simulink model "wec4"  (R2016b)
settings: Solver=ode4  StartTime=0  StopTime=1000  FixedStep=0.005  MaxStep=0.005  RelTol=1e-3  EnableMultiTasking=on
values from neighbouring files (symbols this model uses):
  arAdaptiveLawData = 1/2*zModelSimple.zModelPto.arFreq.*     zModelSimple.zModelPto.arMagnitude./     cos(zModelSimple.zModelPto.arPhase*pi/180+pi/2)    [IMPACT_Control.m]
  arAdaptiveLawDataX = 1/2*zModelSimpleX.zModelPto.arFreq.*         zModelSimpleX.zModelPto.arMagnitude./         cos(zModelSimpleX.zModelPto.arPhase*pi/180+pi/2)    [IMPACT_Control.m]
  arControllerRampGain = [0,0,1,1]    [IMPACT_Control.m]
  arControllerRampTime = [0 rStartRampTime rStartRampTime+rRampTimeLength 8000]    [IMPACT_Control.m]
  arEkfInitialisation = zeros(1,11)    [IMPACT_Control.m]
  arEkfInitialisationX = zeros(1,11)    [IMPACT_Control.m]
  arFrequency = zModelSimple.zModelPto.arFreq    [IMPACT_Control.m]
  arFrequencyRange = zModelSimple.zModelPto.arFreq    [IMPACT_Control.m]
  arFrequencyX = zModelSimpleX.zModelPto.arFreq    [IMPACT_Control.m]
  arImpedance = 1./zModelSimple.zModelPto.arMagnitude./zModelSimple.zModelPto.arFreq    [IMPACT_Control.m]
  arImpedanceX = 1./zModelSimpleX.zModelPto.arMagnitude./zModelSimpleX.zModelPto.arFreq    [IMPACT_Control.m]
  CentralPTOPreload = -1.6113e+07    (= -16113000)    [wecSimInputFile.m]
  F1 = [4.243 2.375 -12.243]    [wecSimInputFile.m]
  F2 = [4.243 -2.375 -12.243]    [wecSimInputFile.m]
  F3 = [-4.243 -2.375 -12.243]    [wecSimInputFile.m]
  F4 = [-4.243 2.375 -12.243]    [wecSimInputFile.m]
  FC = [0 0 -14]    [wecSimInputFile.m]
  iAdaptiveDamping = 0    [wec4IMPACT_Project.m]    (also in IMPACT_Control.m = handles.iAdaptiveDamping; wec1_IMPACT_Project.m; wec2_IMPACT_Project.m; wec3_IMPACT_Project.m)
  iControlType = 2    [wec4IMPACT_Project.m]    (also in IMPACT_Control.m = handles.iControlType; wec1_IMPACT_Project.m = 1; wec2_IMPACT_Project.m = 1; wec3_IMPACT_Project.m = 1)
  iPtoPositionConstraint = 1    [wec4IMPACT_Project.m]    (also in IMPACT_Control.m = handles.iPtoPositionConstraint; wec1_IMPACT_Project.m = 0; wec2_IMPACT_Project.m; wec3_IMPACT_Project.m)
  iSensorNoise = 0    [IMPACT_Control.m]
  m = m+1    (= 2)    [checkParamFile.m]
  PTOrotation = atan((T1(2)-F1(2))/(T1(1)-F1(1)))    [wecSimInputFile.m]
  rCogFloater = -8    [wec4_IMPACT_Model.m]    (also in paramInitial.m = get( handles.edit_rCogFloater, 'String' ); wec1_IMPACT_Model.m = -18; wec2_IMPACT_Model.m = -8.5; wec3_IMPACT_Model.m = -0.7)
  rCogSpar = -36.6    [wec4_IMPACT_Model.m]    (also in paramInitial.m = get( handles.edit_rCogSpar, 'String' ); wec3_IMPACT_Model.m = -21.3; wec3_IMPACT_Model2.m = -21.3)
  rDisplacementLimit = 10.000000    (= 10)    [wec4IMPACT_Project.m]    (also in IMPACT_Control.m = getValue(handles.edit_displacementLimit); wec1_IMPACT_Project.m; wec2_IMPACT_Project.m; wec3_IMPACT_Project.m = 3)
  rDisplacementLimitX = 10.000000    (= 10)    [wec4IMPACT_Project.m]    (also in IMPACT_Control.m = getValue(handles.edit_displacementLimitX); wec1_IMPACT_Project.m = 0; wec2_IMPACT_Project.m; wec3_IMPACT_Project.m = 0)
  rGainForAntiWIndUp = tfControllerDiscrete.rGain    [IMPACT_Control.m]
  rGainForAntiWIndUpX = tfControllerXDiscrete.rGain    [IMPACT_Control.m]
  rMaxForcePto = 300000000.000000    (= 300000000)    [wec4IMPACT_Project.m]    (also in IMPACT_Control.m = getValue(handles.edit_maxForcePto); wec1_IMPACT_Project.m = 1e+15; wec2_IMPACT_Project.m = 1e+15; wec3_IMPACT_Project.m = 1000000000)
  rMinForcePto = -300000000.000000    (= -300000000)    [wec4IMPACT_Project.m]    (also in IMPACT_Control.m = getValue(handles.edit_minForcePto); wec1_IMPACT_Project.m = -1e+15; wec2_IMPACT_Project.m = -1e+15; wec3_IMPACT_Project.m = -1000000000)
  rMooringX = 20000    [wec4_IMPACT_Model.m]    (also in paramInitial.m = get( handles.edit_rMooringX, 'String' ); wec3_IMPACT_Model.m = 10000; wec3_IMPACT_Model2.m = 10000)
  rMooringZ = 10000    [wec4_IMPACT_Model.m]    (also in paramInitial.m = get( handles.edit_rMooringZ, 'String' ); wec3_IMPACT_Model.m = 0; wec3_IMPACT_Model2.m = 0)
  rOutputSampleTime = 0.010000    (= 0.01)    [wec4IMPACT_Project.m]    (also in IMPACT_Control.m = getValue(handles.edit_outputSampleTime); wec1_IMPACT_Project.m; wec2_IMPACT_Project.m; wec3_IMPACT_Project.m)
  rPassiveDampingGain = -604830.000000    (= -604830)    [wec4IMPACT_Project.m]    (also in IMPACT_Control.m = getValue(handles.edit_gainPLD); wec1_IMPACT_Project.m = -214018.1537; wec2_IMPACT_Project.m = -1948070; wec3_IMPACT_Project.m = -519390)
  rPassiveDampingGainX = -278660.000000    (= -278660)    [wec4IMPACT_Project.m]    (also in IMPACT_Control.m = getValue(handles.edit_gainPLDX); wec1_IMPACT_Project.m = 0; wec2_IMPACT_Project.m = 0; wec3_IMPACT_Project.m = 0)
  rTetherPretension = 1.6113e+07    (= 16113000)    [wec4_IMPACT_Model.m]    (also in paramInitial.m = get( handles.edit_rTetherPretension, 'String' ); wec3_IMPACT_Model.m = 0; wec3_IMPACT_Model2.m = 0)
  rTetherSpring = 500000    [wec4_IMPACT_Model.m]    (also in paramInitial.m = get( handles.edit_rTetherSpring, 'String' ); wec3_IMPACT_Model.m = 0; wec3_IMPACT_Model2.m = 0)
  rUpperFrequencyLimit = EKFFloater.upperFreq    [IMPACT_Control.m]
  rXf = 4.243    [wec4AdditionalParams.m]
  rXs = 16.075    [wec4AdditionalParams.m]
  rYf = 2.375    [wec4AdditionalParams.m]
  rYs = 16.075    [wec4AdditionalParams.m]
  rZf = 4.243    [wec4AdditionalParams.m]
  rZs = 2.4350    (= 2.435)    [wec4AdditionalParams.m]
  rZTetherF = 6    [wec4AdditionalParams.m]
  rZTetherS = 2.4350    (= 2.435)    [wec4AdditionalParams.m]
  s = tf('s')    [wec4_IMPACT_Model.m]    (also in IMPACT_Control.m; wec1_IMPACT_Model.m; wec2_IMPACT_Model.m; wec3_IMPACT_Model.m)
  SidePTO1Preload = PreloadPTOCorner    (= 0)    [wecSimInputFile.m]
  SidePTO2Preload = PreloadPTOCorner    (= 0)    [wecSimInputFile.m]
  SidePTO3Preload = PreloadPTOCorner    (= 0)    [wecSimInputFile.m]
  SidePTO4Preload = PreloadPTOCorner    (= 0)    [wecSimInputFile.m]
  simu = simulationClass()    [wecSimInputFile.m]
  T1 = [16.075 16.075 -34.165]    [wecSimInputFile.m]
  T2 = [16.075 -16.075 -34.165]    [wecSimInputFile.m]
  T3 = [-16.075 -16.075 -34.165]    [wecSimInputFile.m]
  T4 = [-16.075 16.075 -34.165]    [wecSimInputFile.m]
  TC = [0 0 -34.165]    [wecSimInputFile.m]
  waves = waveClass('irregular')    [wecSimInputFile.m]
  Z = magPhaseToComplex(zModelTf)    [IMPACT_Control.m]
undefined symbols (not defined in the file or in its folder): arControllerDiscreteDen, arControllerDiscreteNum, arControllerDiscreteXDen, arControllerDiscreteXNum, arExcForceFloaterDen, arExcForceFloaterNum, arExcForceFloaterXDen, arExcForceFloaterXNum, arExcForceSparDen, arExcForceSparNum, arExcForceSparXDen, arExcForceSparXNum, arFexcFloaterDen, arFexcFloaterNum, arFexcFloaterXDen, arFexcFloaterXNum, arFexcSparDen, arFexcSparNum, arFexcSparXDen, arFexcSparXNum, Body, body, constraint, CTTime, deg, Elements, geometry, IRKB, kg, lenJ, mooring, N, pto, rAccelerationGainFloater, rAccelerationGainFloaterX, rAccelerationGainSpar, rAccelerationGainSparX, rad, rBuoyancyGainFloater, rBuoyancyGainFloaterX, rBuoyancyGainSpar, rBuoyancyGainSparX, rDampingGainFloater, rDampingGainFloaterX, rDampingGainSpar, rDampingGainSparX, Rigid, rMaxFocePto, wec4_float, wec4_reactor, WECSim_Lib, X, Y
libraries: nesl_utility x380, sm_lib x170, vrlib x91, simulink x12, WECSim_Lib x4
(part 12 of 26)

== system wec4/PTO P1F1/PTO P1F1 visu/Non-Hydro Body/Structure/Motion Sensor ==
  note: Measures the position, velocity, and acceleration of the follower (F) frame relative to the base (B) frame. Ouputs a bus of 3 signals, each signal is a vector length 6.
  Angle : MATLAB Function  TreatAsAtomicUnit=on
  Bus Creator : BusCreator  Inputs=3
  Mux : Mux
  Mux1 : Mux  Inputs=6
  Mux2 : Mux  Inputs=6
  PS-Simulink Converter{,1..15} (16 alike) : nesl_utility/PS-Simulink Converter  PhysicalDomain=network_engine_domain  SubClassName=ps_output  LeftPortType=input  RightPortType=output  PseudoPeriodic=off  Frequencies=[]  Unit=1  AffineConversion=off
  Transform Sensor : sm_lib/Frames and Transforms/Transform Sensor  MeasurementFrame=World  SenseAngle=off  SenseAxis=off  SenseAngle1=off  SenseAngle2=off  SenseAngle3=off  SenseQ=on  SenseR=off  SenseOmegaX=on  SenseOmegaY=on  SenseOmegaZ=on  SenseOmega1=off  SenseOmega2=off  SenseOmega3=off  SenseQDot=off  SenseRDot=off  SenseAlphaX=on  SenseAlphaY=on  SenseAlphaZ=on  SenseAlpha1=off  SenseAlpha2=off  SenseAlpha3=off  SenseQDDot=off  SenseRDDot=off  SenseX=on  SenseY=on  SenseZ=on  SenseRad=off  SenseAzim=off  SenseDist=off  SenseInc=off  SenseXDot=on  SenseYDot=on  SenseZDot=on  SenseRadDot=off  SenseAzimDot=off  SenseDistDot=off  SenseIncDot=off  SenseXDDot=on  SenseYDDot=on  SenseZDDot=on  SenseRadDDot=off  SenseAzimDDot=off  SenseDistDDot=off  SenseIncDDot=off
  F : PMIOPort  Port=1  Side=Right
  B : PMIOPort  Port=2  Side=Left
  Response : Outport
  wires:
  PS-Simulink Converter/1 -> Angle/1(Q)
  PS-Simulink Converter4/1 -> Mux2/4  "alphax"
  PS-Simulink Converter10/1 -> Mux1/1  "vx"
  PS-Simulink Converter12/1 -> Mux1/3  "vz"
  PS-Simulink Converter13/1 -> Mux2/1  "ax"
  PS-Simulink Converter14/1 -> Mux2/2  "ay"
  Mux/1 -> Bus Creator/1  "disp"
  Mux1/1 -> Bus Creator/2  "vel"
  Mux2/1 -> Bus Creator/3  "acc"
  Angle/1(E) -> Mux/4
  PS-Simulink Converter7/1 -> Mux/1  "x"
  PS-Simulink Converter8/1 -> Mux/2  "y"
  PS-Simulink Converter9/1 -> Mux/3  "z"
  PS-Simulink Converter5/1 -> Mux2/5  "alphay"
  PS-Simulink Converter6/1 -> Mux2/6  "alphaz"
  PS-Simulink Converter1/1 -> Mux1/4  "omegax"
  PS-Simulink Converter2/1 -> Mux1/5  "omegay"
  PS-Simulink Converter11/1 -> Mux1/2  "vy"
  PS-Simulink Converter3/1 -> Mux1/6  "omegaz"
  PS-Simulink Converter15/1 -> Mux2/3  "az"
  Bus Creator/1 -> Response/1
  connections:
  Transform Sensor/RConn1 -- F/RConn1
  B/RConn1 -- Transform Sensor/LConn1
  Transform Sensor/RConn2 -- PS-Simulink Converter/LConn1
  PS-Simulink Converter15/LConn1 -- Transform Sensor/RConn17
  PS-Simulink Converter14/LConn1 -- Transform Sensor/RConn16
  PS-Simulink Converter13/LConn1 -- Transform Sensor/RConn15
  PS-Simulink Converter12/LConn1 -- Transform Sensor/RConn14
  PS-Simulink Converter11/LConn1 -- Transform Sensor/RConn13
  PS-Simulink Converter10/LConn1 -- Transform Sensor/RConn12
  PS-Simulink Converter9/LConn1 -- Transform Sensor/RConn11
  PS-Simulink Converter8/LConn1 -- Transform Sensor/RConn10
  PS-Simulink Converter7/LConn1 -- Transform Sensor/RConn9
  PS-Simulink Converter4/LConn1 -- Transform Sensor/RConn6
  PS-Simulink Converter5/LConn1 -- Transform Sensor/RConn7
  PS-Simulink Converter6/LConn1 -- Transform Sensor/RConn8
  PS-Simulink Converter1/LConn1 -- Transform Sensor/RConn3
  PS-Simulink Converter2/LConn1 -- Transform Sensor/RConn4
  PS-Simulink Converter3/LConn1 -- Transform Sensor/RConn5

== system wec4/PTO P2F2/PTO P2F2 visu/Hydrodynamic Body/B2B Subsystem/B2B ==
  CrossCoupling : Subsystem
  vel : Outport
  acc : Outport  Port=2
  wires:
  CrossCoupling/2(acc) -> acc/1
  CrossCoupling/1(vel) -> vel/1

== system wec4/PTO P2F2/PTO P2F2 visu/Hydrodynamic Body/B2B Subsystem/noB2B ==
  vel_in : Inport
  acc_in : Inport  Port=2
  vel : Outport
  acc : Outport  Port=2
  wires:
  acc_in/1 -> acc/1
  vel_in/1 -> vel/1  "x"

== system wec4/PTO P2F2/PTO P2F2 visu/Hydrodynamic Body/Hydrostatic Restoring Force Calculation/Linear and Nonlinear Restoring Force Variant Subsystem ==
  note: 1) Add Subsystem or Model blocks as valid variant choices. 2) You cannot connect blocks at this level. At simulation, connectivity is automatically determined, based on the active variant and port name matching.
  In1 : Inport
  In2 : Inport  Port=2
  "Linear Hydrostatic Restoring Force " : Subsystem  VariantControl=sv_linearHydro
  Nonlinear Hydrostatic Restoring Force : Subsystem  VariantControl=sv_nonlinearHydro
  Out1 : Outport

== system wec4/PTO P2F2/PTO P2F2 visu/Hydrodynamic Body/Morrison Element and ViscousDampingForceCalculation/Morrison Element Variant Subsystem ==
  note: 1) Add Subsystem or Model blocks as valid variant choices. 2) You cannot connect blocks at this level. At simulation, connectivity is automatically determined, based on the active variant and port name matching.
  displacement : Inport
  velocity : Inport  Port=2
  acceleration : Inport  Port=3
  time : Inport  Port=4
  Morrison Element Off : Subsystem  VariantControl=sv_MEOff
  Morrison Element On : Subsystem  Variant=on  VariantControl=sv_MEOn
  morison_force : Outport

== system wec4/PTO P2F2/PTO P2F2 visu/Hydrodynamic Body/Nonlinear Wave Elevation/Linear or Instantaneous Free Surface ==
  note: 1) Add Subsystem or Model blocks as valid variant choices. 2) You cannot connect blocks at this level. At simulation, connectivity is automatically determined, based on the active variant and port name matching.
  In1 : Inport
  In2 : Inport  Port=2
  "Instantaneous Water Free Surface  " : Subsystem  VariantControl=sv_instFS
  "Mean Water Free Surface " : Subsystem  VariantControl=sv_meanFS
  Out1 : Outport

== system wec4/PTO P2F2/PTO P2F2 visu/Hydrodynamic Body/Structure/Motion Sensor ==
  note: Measures the position, velocity, and acceleration of the follower (F) frame relative to the base (B) frame. Ouputs a bus of 3 signals, each signal is a vector length 6.
  Angle : MATLAB Function  TreatAsAtomicUnit=on
  Bus Creator : BusCreator  Inputs=3
  Mux : Mux
  Mux1 : Mux  Inputs=6
  Mux2 : Mux  Inputs=6
  PS-Simulink Converter{,1..15} (16 alike) : nesl_utility/PS-Simulink Converter  PhysicalDomain=network_engine_domain  SubClassName=ps_output  LeftPortType=input  RightPortType=output  PseudoPeriodic=off  Frequencies=[]  Unit=1  AffineConversion=off
  Transform Sensor : sm_lib/Frames and Transforms/Transform Sensor  MeasurementFrame=World  SenseAngle=off  SenseAxis=off  SenseAngle1=off  SenseAngle2=off  SenseAngle3=off  SenseQ=on  SenseR=off  SenseOmegaX=on  SenseOmegaY=on  SenseOmegaZ=on  SenseOmega1=off  SenseOmega2=off  SenseOmega3=off  SenseQDot=off  SenseRDot=off  SenseAlphaX=on  SenseAlphaY=on  SenseAlphaZ=on  SenseAlpha1=off  SenseAlpha2=off  SenseAlpha3=off  SenseQDDot=off  SenseRDDot=off  SenseX=on  SenseY=on  SenseZ=on  SenseRad=off  SenseAzim=off  SenseDist=off  SenseInc=off  SenseXDot=on  SenseYDot=on  SenseZDot=on  SenseRadDot=off  SenseAzimDot=off  SenseDistDot=off  SenseIncDot=off  SenseXDDot=on  SenseYDDot=on  SenseZDDot=on  SenseRadDDot=off  SenseAzimDDot=off  SenseDistDDot=off  SenseIncDDot=off
  F : PMIOPort  Port=1  Side=Right
  B : PMIOPort  Port=2  Side=Left
  Response : Outport
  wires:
  PS-Simulink Converter/1 -> Angle/1(Q)
  PS-Simulink Converter4/1 -> Mux2/4  "alphax"
  PS-Simulink Converter10/1 -> Mux1/1  "vx"
  PS-Simulink Converter12/1 -> Mux1/3  "vz"
  PS-Simulink Converter13/1 -> Mux2/1  "ax"
  PS-Simulink Converter14/1 -> Mux2/2  "ay"
  Mux/1 -> Bus Creator/1  "disp"
  Mux1/1 -> Bus Creator/2  "vel"
  Mux2/1 -> Bus Creator/3  "acc"
  Angle/1(E) -> Mux/4
  PS-Simulink Converter7/1 -> Mux/1  "x"
  PS-Simulink Converter8/1 -> Mux/2  "y"
  PS-Simulink Converter9/1 -> Mux/3  "z"
  PS-Simulink Converter5/1 -> Mux2/5  "alphay"
  PS-Simulink Converter6/1 -> Mux2/6  "alphaz"
  PS-Simulink Converter1/1 -> Mux1/4  "omegax"
  PS-Simulink Converter2/1 -> Mux1/5  "omegay"
  PS-Simulink Converter11/1 -> Mux1/2  "vy"
  PS-Simulink Converter3/1 -> Mux1/6  "omegaz"
  PS-Simulink Converter15/1 -> Mux2/3  "az"
  Bus Creator/1 -> Response/1
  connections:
  Transform Sensor/RConn1 -- F/RConn1
  B/RConn1 -- Transform Sensor/LConn1
  Transform Sensor/RConn2 -- PS-Simulink Converter/LConn1
  PS-Simulink Converter15/LConn1 -- Transform Sensor/RConn17
  PS-Simulink Converter14/LConn1 -- Transform Sensor/RConn16
  PS-Simulink Converter13/LConn1 -- Transform Sensor/RConn15
  PS-Simulink Converter12/LConn1 -- Transform Sensor/RConn14
  PS-Simulink Converter11/LConn1 -- Transform Sensor/RConn13
  PS-Simulink Converter10/LConn1 -- Transform Sensor/RConn12
  PS-Simulink Converter9/LConn1 -- Transform Sensor/RConn11
  PS-Simulink Converter8/LConn1 -- Transform Sensor/RConn10
  PS-Simulink Converter7/LConn1 -- Transform Sensor/RConn9
  PS-Simulink Converter4/LConn1 -- Transform Sensor/RConn6
  PS-Simulink Converter5/LConn1 -- Transform Sensor/RConn7
  PS-Simulink Converter6/LConn1 -- Transform Sensor/RConn8
  PS-Simulink Converter1/LConn1 -- Transform Sensor/RConn3
  PS-Simulink Converter2/LConn1 -- Transform Sensor/RConn4
  PS-Simulink Converter3/LConn1 -- Transform Sensor/RConn5

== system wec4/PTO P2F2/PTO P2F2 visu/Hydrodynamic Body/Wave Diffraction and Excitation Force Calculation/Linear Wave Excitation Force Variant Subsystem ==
  note: 1) Add Subsystem or Model blocks as valid variant choices. 2) You cannot connect blocks at this level. At simulation, connectivity is automatically determined, based on the active variant and port name matching.
  In1 : Inport
  Irregular Wave Excitation Force : Subsystem  VariantControl=sv_irregularWaves
  No Wave Excitation Force : Subsystem  VariantControl=sv_noWave
  Regular Wave Excitation Force : Subsystem  VariantControl=sv_regularWaves
  User Defined Wave Excitation Force : Subsystem  VariantControl=sv_udfWaves
  Out1 : Outport

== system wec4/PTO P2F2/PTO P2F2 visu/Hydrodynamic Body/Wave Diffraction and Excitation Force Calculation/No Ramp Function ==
  Action Port : ActionPort
  Constant : Constant
  R : Outport  InitialOutput=1
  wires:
  Constant/1 -> R/1

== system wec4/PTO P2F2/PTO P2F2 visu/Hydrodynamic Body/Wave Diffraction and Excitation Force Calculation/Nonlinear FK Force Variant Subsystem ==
  note: 1) Add Subsystem or Model blocks as valid variant choices. 2) You cannot connect blocks at this level. At simulation, connectivity is automatically determined, based on the active variant and port name matching.
  In1 : Inport
  In2 : Inport  Port=2
  In3 : Inport  Port=3
  No Nonlinear FroudeKrylov Force : Subsystem  VariantControl=sv_linearHydro
  With Nonlinear FroudeKrylov Force : Subsystem  TreatAsAtomicUnit=on  SystemSampleTime=simu.dtNL  VariantControl=sv_nonlinearHydro
  Out1 : Outport

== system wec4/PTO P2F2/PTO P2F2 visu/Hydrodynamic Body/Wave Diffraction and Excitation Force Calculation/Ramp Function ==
  Time : Inport
  Action Port : ActionPort
  Add : Sum
  Add1 : Sum
  Constant : Constant  Value=1/2
  Constant1 : Constant
  Constant2 : Constant  Value=3*pi/2
  Constant3 : Constant  Value=pi
  Divide : Product  Inputs=*/
  Product : Product
  Product1 : Product
  Ramp Time : Constant  Value=simu.rampTime
  Sine Wave Function : Sin  TimeSource=Use external signal  SampleTime=0
  R : Outport
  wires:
  Divide/1 -> Product1/2  "frequency"
  Constant3/1 -> Divide/1
  Product1/1 -> Add1/1
  Add1/1 -> Sine Wave Function/1
  Constant2/1 -> Add1/2  "phase"
  Ramp Time/1 -> Divide/2  "t_ramp"
  Time/1 -> Product1/1  "t"
  Product/1 -> R/1
  Constant/1 -> Product/2
  Constant1/1 -> Add/1
  Sine Wave Function/1 -> Add/2
  Add/1 -> Product/1

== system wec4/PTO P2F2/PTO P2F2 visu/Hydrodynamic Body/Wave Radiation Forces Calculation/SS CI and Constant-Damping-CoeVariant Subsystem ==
  note: 1) Add Subsystem or Model blocks as valid variant choices. 2) You cannot connect blocks at this level. At simulation, connectivity is automatically determined, based on the active variant and port name matching.
  In1 : Inport
  In2 : Inport  Port=2
  Constant Coefficients : Subsystem  VariantControl=sv_constantCoeff
  Convolution Integral Calculation : Subsystem  VariantControl=sv_convolution
  "State-Space Calculation " : Subsystem  VariantControl=sv_stateSpace
  Out1 : Outport

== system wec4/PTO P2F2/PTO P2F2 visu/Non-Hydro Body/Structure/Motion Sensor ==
  note: Measures the position, velocity, and acceleration of the follower (F) frame relative to the base (B) frame. Ouputs a bus of 3 signals, each signal is a vector length 6.
  Angle : MATLAB Function  TreatAsAtomicUnit=on
  Bus Creator : BusCreator  Inputs=3
  Mux : Mux
  Mux1 : Mux  Inputs=6
  Mux2 : Mux  Inputs=6
  PS-Simulink Converter{,1..15} (16 alike) : nesl_utility/PS-Simulink Converter  PhysicalDomain=network_engine_domain  SubClassName=ps_output  LeftPortType=input  RightPortType=output  PseudoPeriodic=off  Frequencies=[]  Unit=1  AffineConversion=off
  Transform Sensor : sm_lib/Frames and Transforms/Transform Sensor  MeasurementFrame=World  SenseAngle=off  SenseAxis=off  SenseAngle1=off  SenseAngle2=off  SenseAngle3=off  SenseQ=on  SenseR=off  SenseOmegaX=on  SenseOmegaY=on  SenseOmegaZ=on  SenseOmega1=off  SenseOmega2=off  SenseOmega3=off  SenseQDot=off  SenseRDot=off  SenseAlphaX=on  SenseAlphaY=on  SenseAlphaZ=on  SenseAlpha1=off  SenseAlpha2=off  SenseAlpha3=off  SenseQDDot=off  SenseRDDot=off  SenseX=on  SenseY=on  SenseZ=on  SenseRad=off  SenseAzim=off  SenseDist=off  SenseInc=off  SenseXDot=on  SenseYDot=on  SenseZDot=on  SenseRadDot=off  SenseAzimDot=off  SenseDistDot=off  SenseIncDot=off  SenseXDDot=on  SenseYDDot=on  SenseZDDot=on  SenseRadDDot=off  SenseAzimDDot=off  SenseDistDDot=off  SenseIncDDot=off
  F : PMIOPort  Port=1  Side=Right
  B : PMIOPort  Port=2  Side=Left
  Response : Outport
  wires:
  PS-Simulink Converter/1 -> Angle/1(Q)
  PS-Simulink Converter4/1 -> Mux2/4  "alphax"
  PS-Simulink Converter10/1 -> Mux1/1  "vx"
  PS-Simulink Converter12/1 -> Mux1/3  "vz"
  PS-Simulink Converter13/1 -> Mux2/1  "ax"
  PS-Simulink Converter14/1 -> Mux2/2  "ay"
  Mux/1 -> Bus Creator/1  "disp"
  Mux1/1 -> Bus Creator/2  "vel"
  Mux2/1 -> Bus Creator/3  "acc"
  Angle/1(E) -> Mux/4
  PS-Simulink Converter7/1 -> Mux/1  "x"
  PS-Simulink Converter8/1 -> Mux/2  "y"
  PS-Simulink Converter9/1 -> Mux/3  "z"
  PS-Simulink Converter5/1 -> Mux2/5  "alphay"
  PS-Simulink Converter6/1 -> Mux2/6  "alphaz"
  PS-Simulink Converter1/1 -> Mux1/4  "omegax"
  PS-Simulink Converter2/1 -> Mux1/5  "omegay"
  PS-Simulink Converter11/1 -> Mux1/2  "vy"
  PS-Simulink Converter3/1 -> Mux1/6  "omegaz"
  PS-Simulink Converter15/1 -> Mux2/3  "az"
  Bus Creator/1 -> Response/1
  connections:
  Transform Sensor/RConn1 -- F/RConn1
  B/RConn1 -- Transform Sensor/LConn1
  Transform Sensor/RConn2 -- PS-Simulink Converter/LConn1
  PS-Simulink Converter15/LConn1 -- Transform Sensor/RConn17
  PS-Simulink Converter14/LConn1 -- Transform Sensor/RConn16
  PS-Simulink Converter13/LConn1 -- Transform Sensor/RConn15
  PS-Simulink Converter12/LConn1 -- Transform Sensor/RConn14
  PS-Simulink Converter11/LConn1 -- Transform Sensor/RConn13
  PS-Simulink Converter10/LConn1 -- Transform Sensor/RConn12
  PS-Simulink Converter9/LConn1 -- Transform Sensor/RConn11
  PS-Simulink Converter8/LConn1 -- Transform Sensor/RConn10
  PS-Simulink Converter7/LConn1 -- Transform Sensor/RConn9
  PS-Simulink Converter4/LConn1 -- Transform Sensor/RConn6
  PS-Simulink Converter5/LConn1 -- Transform Sensor/RConn7
  PS-Simulink Converter6/LConn1 -- Transform Sensor/RConn8
  PS-Simulink Converter1/LConn1 -- Transform Sensor/RConn3
  PS-Simulink Converter2/LConn1 -- Transform Sensor/RConn4
  PS-Simulink Converter3/LConn1 -- Transform Sensor/RConn5

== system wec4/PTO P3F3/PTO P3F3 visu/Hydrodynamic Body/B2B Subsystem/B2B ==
  CrossCoupling : Subsystem
  vel : Outport
  acc : Outport  Port=2
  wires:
  CrossCoupling/2(acc) -> acc/1
  CrossCoupling/1(vel) -> vel/1

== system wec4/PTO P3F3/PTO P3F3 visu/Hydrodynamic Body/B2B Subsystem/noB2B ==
  vel_in : Inport
  acc_in : Inport  Port=2
  vel : Outport
  acc : Outport  Port=2
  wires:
  acc_in/1 -> acc/1
  vel_in/1 -> vel/1  "x"

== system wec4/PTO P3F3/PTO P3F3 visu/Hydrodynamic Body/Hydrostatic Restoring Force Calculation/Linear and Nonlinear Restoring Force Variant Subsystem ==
  note: 1) Add Subsystem or Model blocks as valid variant choices. 2) You cannot connect blocks at this level. At simulation, connectivity is automatically determined, based on the active variant and port name matching.
  In1 : Inport
  In2 : Inport  Port=2
  "Linear Hydrostatic Restoring Force " : Subsystem  VariantControl=sv_linearHydro
  Nonlinear Hydrostatic Restoring Force : Subsystem  VariantControl=sv_nonlinearHydro
  Out1 : Outport

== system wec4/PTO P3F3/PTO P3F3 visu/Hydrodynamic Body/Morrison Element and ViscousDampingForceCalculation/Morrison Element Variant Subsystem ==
  note: 1) Add Subsystem or Model blocks as valid variant choices. 2) You cannot connect blocks at this level. At simulation, connectivity is automatically determined, based on the active variant and port name matching.
  displacement : Inport
  velocity : Inport  Port=2
  acceleration : Inport  Port=3
  time : Inport  Port=4
  Morrison Element Off : Subsystem  VariantControl=sv_MEOff
  Morrison Element On : Subsystem  Variant=on  VariantControl=sv_MEOn
  morison_force : Outport

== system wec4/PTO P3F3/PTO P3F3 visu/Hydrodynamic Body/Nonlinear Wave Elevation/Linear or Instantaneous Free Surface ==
  note: 1) Add Subsystem or Model blocks as valid variant choices. 2) You cannot connect blocks at this level. At simulation, connectivity is automatically determined, based on the active variant and port name matching.
  In1 : Inport
  In2 : Inport  Port=2
  "Instantaneous Water Free Surface  " : Subsystem  VariantControl=sv_instFS
  "Mean Water Free Surface " : Subsystem  VariantControl=sv_meanFS
  Out1 : Outport

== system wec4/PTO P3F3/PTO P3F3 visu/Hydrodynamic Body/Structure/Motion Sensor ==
  note: Measures the position, velocity, and acceleration of the follower (F) frame relative to the base (B) frame. Ouputs a bus of 3 signals, each signal is a vector length 6.
  Angle : MATLAB Function  TreatAsAtomicUnit=on
  Bus Creator : BusCreator  Inputs=3
  Mux : Mux
  Mux1 : Mux  Inputs=6
  Mux2 : Mux  Inputs=6
  PS-Simulink Converter{,1..15} (16 alike) : nesl_utility/PS-Simulink Converter  PhysicalDomain=network_engine_domain  SubClassName=ps_output  LeftPortType=input  RightPortType=output  PseudoPeriodic=off  Frequencies=[]  Unit=1  AffineConversion=off
  Transform Sensor : sm_lib/Frames and Transforms/Transform Sensor  MeasurementFrame=World  SenseAngle=off  SenseAxis=off  SenseAngle1=off  SenseAngle2=off  SenseAngle3=off  SenseQ=on  SenseR=off  SenseOmegaX=on  SenseOmegaY=on  SenseOmegaZ=on  SenseOmega1=off  SenseOmega2=off  SenseOmega3=off  SenseQDot=off  SenseRDot=off  SenseAlphaX=on  SenseAlphaY=on  SenseAlphaZ=on  SenseAlpha1=off  SenseAlpha2=off  SenseAlpha3=off  SenseQDDot=off  SenseRDDot=off  SenseX=on  SenseY=on  SenseZ=on  SenseRad=off  SenseAzim=off  SenseDist=off  SenseInc=off  SenseXDot=on  SenseYDot=on  SenseZDot=on  SenseRadDot=off  SenseAzimDot=off  SenseDistDot=off  SenseIncDot=off  SenseXDDot=on  SenseYDDot=on  SenseZDDot=on  SenseRadDDot=off  SenseAzimDDot=off  SenseDistDDot=off  SenseIncDDot=off
  F : PMIOPort  Port=1  Side=Right
  B : PMIOPort  Port=2  Side=Left
  Response : Outport
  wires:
  PS-Simulink Converter/1 -> Angle/1(Q)
  PS-Simulink Converter4/1 -> Mux2/4  "alphax"
  PS-Simulink Converter10/1 -> Mux1/1  "vx"
  PS-Simulink Converter12/1 -> Mux1/3  "vz"
  PS-Simulink Converter13/1 -> Mux2/1  "ax"
  PS-Simulink Converter14/1 -> Mux2/2  "ay"
  Mux/1 -> Bus Creator/1  "disp"
  Mux1/1 -> Bus Creator/2  "vel"
  Mux2/1 -> Bus Creator/3  "acc"
  Angle/1(E) -> Mux/4
  PS-Simulink Converter7/1 -> Mux/1  "x"
  PS-Simulink Converter8/1 -> Mux/2  "y"
  PS-Simulink Converter9/1 -> Mux/3  "z"
  PS-Simulink Converter5/1 -> Mux2/5  "alphay"
  PS-Simulink Converter6/1 -> Mux2/6  "alphaz"
  PS-Simulink Converter1/1 -> Mux1/4  "omegax"
  PS-Simulink Converter2/1 -> Mux1/5  "omegay"
  PS-Simulink Converter11/1 -> Mux1/2  "vy"
  PS-Simulink Converter3/1 -> Mux1/6  "omegaz"
  PS-Simulink Converter15/1 -> Mux2/3  "az"
  Bus Creator/1 -> Response/1
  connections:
  Transform Sensor/RConn1 -- F/RConn1
  B/RConn1 -- Transform Sensor/LConn1
  Transform Sensor/RConn2 -- PS-Simulink Converter/LConn1
  PS-Simulink Converter15/LConn1 -- Transform Sensor/RConn17
  PS-Simulink Converter14/LConn1 -- Transform Sensor/RConn16
  PS-Simulink Converter13/LConn1 -- Transform Sensor/RConn15
  PS-Simulink Converter12/LConn1 -- Transform Sensor/RConn14
  PS-Simulink Converter11/LConn1 -- Transform Sensor/RConn13
  PS-Simulink Converter10/LConn1 -- Transform Sensor/RConn12
  PS-Simulink Converter9/LConn1 -- Transform Sensor/RConn11
  PS-Simulink Converter8/LConn1 -- Transform Sensor/RConn10
  PS-Simulink Converter7/LConn1 -- Transform Sensor/RConn9
  PS-Simulink Converter4/LConn1 -- Transform Sensor/RConn6
  PS-Simulink Converter5/LConn1 -- Transform Sensor/RConn7
  PS-Simulink Converter6/LConn1 -- Transform Sensor/RConn8
  PS-Simulink Converter1/LConn1 -- Transform Sensor/RConn3
  PS-Simulink Converter2/LConn1 -- Transform Sensor/RConn4
  PS-Simulink Converter3/LConn1 -- Transform Sensor/RConn5

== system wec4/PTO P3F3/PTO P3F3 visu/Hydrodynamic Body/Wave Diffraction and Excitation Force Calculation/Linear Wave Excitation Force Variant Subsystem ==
  note: 1) Add Subsystem or Model blocks as valid variant choices. 2) You cannot connect blocks at this level. At simulation, connectivity is automatically determined, based on the active variant and port name matching.
  In1 : Inport
  Irregular Wave Excitation Force : Subsystem  VariantControl=sv_irregularWaves
  No Wave Excitation Force : Subsystem  VariantControl=sv_noWave
  Regular Wave Excitation Force : Subsystem  VariantControl=sv_regularWaves
  User Defined Wave Excitation Force : Subsystem  VariantControl=sv_udfWaves
  Out1 : Outport

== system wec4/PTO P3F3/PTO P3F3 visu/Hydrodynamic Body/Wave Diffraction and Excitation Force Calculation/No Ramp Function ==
  Action Port : ActionPort
  Constant : Constant
  R : Outport  InitialOutput=1
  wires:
  Constant/1 -> R/1

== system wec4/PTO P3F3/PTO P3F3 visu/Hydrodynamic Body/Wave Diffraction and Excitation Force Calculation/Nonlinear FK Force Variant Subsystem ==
  note: 1) Add Subsystem or Model blocks as valid variant choices. 2) You cannot connect blocks at this level. At simulation, connectivity is automatically determined, based on the active variant and port name matching.
  In1 : Inport
  In2 : Inport  Port=2
  In3 : Inport  Port=3
  No Nonlinear FroudeKrylov Force : Subsystem  VariantControl=sv_linearHydro
  With Nonlinear FroudeKrylov Force : Subsystem  TreatAsAtomicUnit=on  SystemSampleTime=simu.dtNL  VariantControl=sv_nonlinearHydro
  Out1 : Outport

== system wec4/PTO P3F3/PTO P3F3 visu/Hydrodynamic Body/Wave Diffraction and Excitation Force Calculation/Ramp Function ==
  Time : Inport
  Action Port : ActionPort
  Add : Sum
  Add1 : Sum
  Constant : Constant  Value=1/2
  Constant1 : Constant
  Constant2 : Constant  Value=3*pi/2
  Constant3 : Constant  Value=pi
  Divide : Product  Inputs=*/
  Product : Product
  Product1 : Product
  Ramp Time : Constant  Value=simu.rampTime
  Sine Wave Function : Sin  TimeSource=Use external signal  SampleTime=0
  R : Outport
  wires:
  Divide/1 -> Product1/2  "frequency"
  Constant3/1 -> Divide/1
  Product1/1 -> Add1/1
  Add1/1 -> Sine Wave Function/1
  Constant2/1 -> Add1/2  "phase"
  Ramp Time/1 -> Divide/2  "t_ramp"
  Time/1 -> Product1/1  "t"
  Product/1 -> R/1
  Constant/1 -> Product/2
  Constant1/1 -> Add/1
  Sine Wave Function/1 -> Add/2
  Add/1 -> Product/1

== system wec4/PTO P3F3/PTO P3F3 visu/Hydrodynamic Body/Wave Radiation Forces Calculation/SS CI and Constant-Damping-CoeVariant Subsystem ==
  note: 1) Add Subsystem or Model blocks as valid variant choices. 2) You cannot connect blocks at this level. At simulation, connectivity is automatically determined, based on the active variant and port name matching.
  In1 : Inport
  In2 : Inport  Port=2
  Constant Coefficients : Subsystem  VariantControl=sv_constantCoeff
  Convolution Integral Calculation : Subsystem  VariantControl=sv_convolution
  "State-Space Calculation " : Subsystem  VariantControl=sv_stateSpace
  Out1 : Outport

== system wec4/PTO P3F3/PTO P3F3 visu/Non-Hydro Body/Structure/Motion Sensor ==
  note: Measures the position, velocity, and acceleration of the follower (F) frame relative to the base (B) frame. Ouputs a bus of 3 signals, each signal is a vector length 6.
  Angle : MATLAB Function  TreatAsAtomicUnit=on
  Bus Creator : BusCreator  Inputs=3
  Mux : Mux
  Mux1 : Mux  Inputs=6
  Mux2 : Mux  Inputs=6
  PS-Simulink Converter{,1..15} (16 alike) : nesl_utility/PS-Simulink Converter  PhysicalDomain=network_engine_domain  SubClassName=ps_output  LeftPortType=input  RightPortType=output  PseudoPeriodic=off  Frequencies=[]  Unit=1  AffineConversion=off
  Transform Sensor : sm_lib/Frames and Transforms/Transform Sensor  MeasurementFrame=World  SenseAngle=off  SenseAxis=off  SenseAngle1=off  SenseAngle2=off  SenseAngle3=off  SenseQ=on  SenseR=off  SenseOmegaX=on  SenseOmegaY=on  SenseOmegaZ=on  SenseOmega1=off  SenseOmega2=off  SenseOmega3=off  SenseQDot=off  SenseRDot=off  SenseAlphaX=on  SenseAlphaY=on  SenseAlphaZ=on  SenseAlpha1=off  SenseAlpha2=off  SenseAlpha3=off  SenseQDDot=off  SenseRDDot=off  SenseX=on  SenseY=on  SenseZ=on  SenseRad=off  SenseAzim=off  SenseDist=off  SenseInc=off  SenseXDot=on  SenseYDot=on  SenseZDot=on  SenseRadDot=off  SenseAzimDot=off  SenseDistDot=off  SenseIncDot=off  SenseXDDot=on  SenseYDDot=on  SenseZDDot=on  SenseRadDDot=off  SenseAzimDDot=off  SenseDistDDot=off  SenseIncDDot=off
  F : PMIOPort  Port=1  Side=Right
  B : PMIOPort  Port=2  Side=Left
  Response : Outport
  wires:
  PS-Simulink Converter/1 -> Angle/1(Q)
  PS-Simulink Converter4/1 -> Mux2/4  "alphax"
  PS-Simulink Converter10/1 -> Mux1/1  "vx"
  PS-Simulink Converter12/1 -> Mux1/3  "vz"
  PS-Simulink Converter13/1 -> Mux2/1  "ax"
  PS-Simulink Converter14/1 -> Mux2/2  "ay"
  Mux/1 -> Bus Creator/1  "disp"
  Mux1/1 -> Bus Creator/2  "vel"
  Mux2/1 -> Bus Creator/3  "acc"
  Angle/1(E) -> Mux/4
  PS-Simulink Converter7/1 -> Mux/1  "x"
  PS-Simulink Converter8/1 -> Mux/2  "y"
  PS-Simulink Converter9/1 -> Mux/3  "z"
  PS-Simulink Converter5/1 -> Mux2/5  "alphay"
  PS-Simulink Converter6/1 -> Mux2/6  "alphaz"
  PS-Simulink Converter1/1 -> Mux1/4  "omegax"
  PS-Simulink Converter2/1 -> Mux1/5  "omegay"
  PS-Simulink Converter11/1 -> Mux1/2  "vy"
  PS-Simulink Converter3/1 -> Mux1/6  "omegaz"
  PS-Simulink Converter15/1 -> Mux2/3  "az"
  Bus Creator/1 -> Response/1
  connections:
  Transform Sensor/RConn1 -- F/RConn1
  B/RConn1 -- Transform Sensor/LConn1
  Transform Sensor/RConn2 -- PS-Simulink Converter/LConn1
  PS-Simulink Converter15/LConn1 -- Transform Sensor/RConn17
  PS-Simulink Converter14/LConn1 -- Transform Sensor/RConn16
  PS-Simulink Converter13/LConn1 -- Transform Sensor/RConn15
  PS-Simulink Converter12/LConn1 -- Transform Sensor/RConn14
  PS-Simulink Converter11/LConn1 -- Transform Sensor/RConn13
  PS-Simulink Converter10/LConn1 -- Transform Sensor/RConn12
  PS-Simulink Converter9/LConn1 -- Transform Sensor/RConn11
  PS-Simulink Converter8/LConn1 -- Transform Sensor/RConn10
  PS-Simulink Converter7/LConn1 -- Transform Sensor/RConn9
  PS-Simulink Converter4/LConn1 -- Transform Sensor/RConn6
  PS-Simulink Converter5/LConn1 -- Transform Sensor/RConn7
  PS-Simulink Converter6/LConn1 -- Transform Sensor/RConn8
  PS-Simulink Converter1/LConn1 -- Transform Sensor/RConn3
  PS-Simulink Converter2/LConn1 -- Transform Sensor/RConn4
  PS-Simulink Converter3/LConn1 -- Transform Sensor/RConn5

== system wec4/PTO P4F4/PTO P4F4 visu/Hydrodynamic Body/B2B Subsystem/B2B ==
  CrossCoupling : Subsystem
  vel : Outport
  acc : Outport  Port=2
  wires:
  CrossCoupling/2(acc) -> acc/1
  CrossCoupling/1(vel) -> vel/1

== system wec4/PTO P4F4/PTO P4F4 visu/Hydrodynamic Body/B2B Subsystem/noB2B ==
  vel_in : Inport
  acc_in : Inport  Port=2
  vel : Outport
  acc : Outport  Port=2
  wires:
  acc_in/1 -> acc/1
  vel_in/1 -> vel/1  "x"

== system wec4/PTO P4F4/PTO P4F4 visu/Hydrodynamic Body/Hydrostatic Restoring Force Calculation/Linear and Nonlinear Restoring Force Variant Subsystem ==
  note: 1) Add Subsystem or Model blocks as valid variant choices. 2) You cannot connect blocks at this level. At simulation, connectivity is automatically determined, based on the active variant and port name matching.
  In1 : Inport
  In2 : Inport  Port=2
  "Linear Hydrostatic Restoring Force " : Subsystem  VariantControl=sv_linearHydro
  Nonlinear Hydrostatic Restoring Force : Subsystem  VariantControl=sv_nonlinearHydro
  Out1 : Outport

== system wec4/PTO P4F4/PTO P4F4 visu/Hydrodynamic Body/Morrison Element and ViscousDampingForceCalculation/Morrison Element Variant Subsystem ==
  note: 1) Add Subsystem or Model blocks as valid variant choices. 2) You cannot connect blocks at this level. At simulation, connectivity is automatically determined, based on the active variant and port name matching.
  displacement : Inport
  velocity : Inport  Port=2
  acceleration : Inport  Port=3
  time : Inport  Port=4
  Morrison Element Off : Subsystem  VariantControl=sv_MEOff
  Morrison Element On : Subsystem  Variant=on  VariantControl=sv_MEOn
  morison_force : Outport

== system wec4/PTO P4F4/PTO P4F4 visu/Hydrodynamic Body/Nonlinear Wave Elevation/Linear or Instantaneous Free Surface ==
  note: 1) Add Subsystem or Model blocks as valid variant choices. 2) You cannot connect blocks at this level. At simulation, connectivity is automatically determined, based on the active variant and port name matching.
  In1 : Inport
  In2 : Inport  Port=2
  "Instantaneous Water Free Surface  " : Subsystem  VariantControl=sv_instFS
  "Mean Water Free Surface " : Subsystem  VariantControl=sv_meanFS
  Out1 : Outport

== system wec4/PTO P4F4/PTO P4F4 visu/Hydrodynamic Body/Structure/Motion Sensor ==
  note: Measures the position, velocity, and acceleration of the follower (F) frame relative to the base (B) frame. Ouputs a bus of 3 signals, each signal is a vector length 6.
  Angle : MATLAB Function  TreatAsAtomicUnit=on
  Bus Creator : BusCreator  Inputs=3
  Mux : Mux
  Mux1 : Mux  Inputs=6
  Mux2 : Mux  Inputs=6
  PS-Simulink Converter{,1..15} (16 alike) : nesl_utility/PS-Simulink Converter  PhysicalDomain=network_engine_domain  SubClassName=ps_output  LeftPortType=input  RightPortType=output  PseudoPeriodic=off  Frequencies=[]  Unit=1  AffineConversion=off
  Transform Sensor : sm_lib/Frames and Transforms/Transform Sensor  MeasurementFrame=World  SenseAngle=off  SenseAxis=off  SenseAngle1=off  SenseAngle2=off  SenseAngle3=off  SenseQ=on  SenseR=off  SenseOmegaX=on  SenseOmegaY=on  SenseOmegaZ=on  SenseOmega1=off  SenseOmega2=off  SenseOmega3=off  SenseQDot=off  SenseRDot=off  SenseAlphaX=on  SenseAlphaY=on  SenseAlphaZ=on  SenseAlpha1=off  SenseAlpha2=off  SenseAlpha3=off  SenseQDDot=off  SenseRDDot=off  SenseX=on  SenseY=on  SenseZ=on  SenseRad=off  SenseAzim=off  SenseDist=off  SenseInc=off  SenseXDot=on  SenseYDot=on  SenseZDot=on  SenseRadDot=off  SenseAzimDot=off  SenseDistDot=off  SenseIncDot=off  SenseXDDot=on  SenseYDDot=on  SenseZDDot=on  SenseRadDDot=off  SenseAzimDDot=off  SenseDistDDot=off  SenseIncDDot=off
  F : PMIOPort  Port=1  Side=Right
  B : PMIOPort  Port=2  Side=Left
  Response : Outport
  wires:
  PS-Simulink Converter/1 -> Angle/1(Q)
  PS-Simulink Converter4/1 -> Mux2/4  "alphax"
  PS-Simulink Converter10/1 -> Mux1/1  "vx"
  PS-Simulink Converter12/1 -> Mux1/3  "vz"
  PS-Simulink Converter13/1 -> Mux2/1  "ax"
  PS-Simulink Converter14/1 -> Mux2/2  "ay"
  Mux/1 -> Bus Creator/1  "disp"
  Mux1/1 -> Bus Creator/2  "vel"
  Mux2/1 -> Bus Creator/3  "acc"
  Angle/1(E) -> Mux/4
  PS-Simulink Converter7/1 -> Mux/1  "x"
  PS-Simulink Converter8/1 -> Mux/2  "y"
  PS-Simulink Converter9/1 -> Mux/3  "z"
  PS-Simulink Converter5/1 -> Mux2/5  "alphay"
  PS-Simulink Converter6/1 -> Mux2/6  "alphaz"
  PS-Simulink Converter1/1 -> Mux1/4  "omegax"
  PS-Simulink Converter2/1 -> Mux1/5  "omegay"
  PS-Simulink Converter11/1 -> Mux1/2  "vy"
  PS-Simulink Converter3/1 -> Mux1/6  "omegaz"
  PS-Simulink Converter15/1 -> Mux2/3  "az"
  Bus Creator/1 -> Response/1
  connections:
  Transform Sensor/RConn1 -- F/RConn1
  B/RConn1 -- Transform Sensor/LConn1
  Transform Sensor/RConn2 -- PS-Simulink Converter/LConn1
  PS-Simulink Converter15/LConn1 -- Transform Sensor/RConn17
  PS-Simulink Converter14/LConn1 -- Transform Sensor/RConn16
  PS-Simulink Converter13/LConn1 -- Transform Sensor/RConn15
  PS-Simulink Converter12/LConn1 -- Transform Sensor/RConn14
  PS-Simulink Converter11/LConn1 -- Transform Sensor/RConn13
  PS-Simulink Converter10/LConn1 -- Transform Sensor/RConn12
  PS-Simulink Converter9/LConn1 -- Transform Sensor/RConn11
  PS-Simulink Converter8/LConn1 -- Transform Sensor/RConn10
  PS-Simulink Converter7/LConn1 -- Transform Sensor/RConn9
  PS-Simulink Converter4/LConn1 -- Transform Sensor/RConn6
  PS-Simulink Converter5/LConn1 -- Transform Sensor/RConn7
  PS-Simulink Converter6/LConn1 -- Transform Sensor/RConn8
  PS-Simulink Converter1/LConn1 -- Transform Sensor/RConn3
  PS-Simulink Converter2/LConn1 -- Transform Sensor/RConn4
  PS-Simulink Converter3/LConn1 -- Transform Sensor/RConn5

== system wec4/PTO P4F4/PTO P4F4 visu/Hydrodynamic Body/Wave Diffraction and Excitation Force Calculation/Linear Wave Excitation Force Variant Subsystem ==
  note: 1) Add Subsystem or Model blocks as valid variant choices. 2) You cannot connect blocks at this level. At simulation, connectivity is automatically determined, based on the active variant and port name matching.
  In1 : Inport
  Irregular Wave Excitation Force : Subsystem  VariantControl=sv_irregularWaves
  No Wave Excitation Force : Subsystem  VariantControl=sv_noWave
  Regular Wave Excitation Force : Subsystem  VariantControl=sv_regularWaves
  User Defined Wave Excitation Force : Subsystem  VariantControl=sv_udfWaves
  Out1 : Outport

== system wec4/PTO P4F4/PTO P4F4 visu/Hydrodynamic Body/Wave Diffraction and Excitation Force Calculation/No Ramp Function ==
  Action Port : ActionPort
  Constant : Constant
  R : Outport  InitialOutput=1
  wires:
  Constant/1 -> R/1

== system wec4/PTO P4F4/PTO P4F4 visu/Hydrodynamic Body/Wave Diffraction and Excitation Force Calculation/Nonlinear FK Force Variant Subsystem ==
  note: 1) Add Subsystem or Model blocks as valid variant choices. 2) You cannot connect blocks at this level. At simulation, connectivity is automatically determined, based on the active variant and port name matching.
  In1 : Inport
  In2 : Inport  Port=2
  In3 : Inport  Port=3
  No Nonlinear FroudeKrylov Force : Subsystem  VariantControl=sv_linearHydro
  With Nonlinear FroudeKrylov Force : Subsystem  TreatAsAtomicUnit=on  SystemSampleTime=simu.dtNL  VariantControl=sv_nonlinearHydro
  Out1 : Outport

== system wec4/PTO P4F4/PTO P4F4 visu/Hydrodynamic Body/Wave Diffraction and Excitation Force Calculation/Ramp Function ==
  Time : Inport
  Action Port : ActionPort
  Add : Sum
  Add1 : Sum
  Constant : Constant  Value=1/2
  Constant1 : Constant
  Constant2 : Constant  Value=3*pi/2
  Constant3 : Constant  Value=pi
  Divide : Product  Inputs=*/
  Product : Product
  Product1 : Product
  Ramp Time : Constant  Value=simu.rampTime
  Sine Wave Function : Sin  TimeSource=Use external signal  SampleTime=0
  R : Outport
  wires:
  Divide/1 -> Product1/2  "frequency"
  Constant3/1 -> Divide/1
  Product1/1 -> Add1/1
  Add1/1 -> Sine Wave Function/1
  Constant2/1 -> Add1/2  "phase"
  Ramp Time/1 -> Divide/2  "t_ramp"
  Time/1 -> Product1/1  "t"
  Product/1 -> R/1
  Constant/1 -> Product/2
  Constant1/1 -> Add/1
  Sine Wave Function/1 -> Add/2
  Add/1 -> Product/1

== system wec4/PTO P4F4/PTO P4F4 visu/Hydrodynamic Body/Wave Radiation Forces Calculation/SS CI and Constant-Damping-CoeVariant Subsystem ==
  note: 1) Add Subsystem or Model blocks as valid variant choices. 2) You cannot connect blocks at this level. At simulation, connectivity is automatically determined, based on the active variant and port name matching.
  In1 : Inport
  In2 : Inport  Port=2
  Constant Coefficients : Subsystem  VariantControl=sv_constantCoeff
  Convolution Integral Calculation : Subsystem  VariantControl=sv_convolution
  "State-Space Calculation " : Subsystem  VariantControl=sv_stateSpace
  Out1 : Outport

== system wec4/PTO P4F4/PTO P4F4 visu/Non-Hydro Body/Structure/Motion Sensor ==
  note: Measures the position, velocity, and acceleration of the follower (F) frame relative to the base (B) frame. Ouputs a bus of 3 signals, each signal is a vector length 6.
  Angle : MATLAB Function  TreatAsAtomicUnit=on
  Bus Creator : BusCreator  Inputs=3
  Mux : Mux
  Mux1 : Mux  Inputs=6
  Mux2 : Mux  Inputs=6
  PS-Simulink Converter{,1..15} (16 alike) : nesl_utility/PS-Simulink Converter  PhysicalDomain=network_engine_domain  SubClassName=ps_output  LeftPortType=input  RightPortType=output  PseudoPeriodic=off  Frequencies=[]  Unit=1  AffineConversion=off
  Transform Sensor : sm_lib/Frames and Transforms/Transform Sensor  MeasurementFrame=World  SenseAngle=off  SenseAxis=off  SenseAngle1=off  SenseAngle2=off  SenseAngle3=off  SenseQ=on  SenseR=off  SenseOmegaX=on  SenseOmegaY=on  SenseOmegaZ=on  SenseOmega1=off  SenseOmega2=off  SenseOmega3=off  SenseQDot=off  SenseRDot=off  SenseAlphaX=on  SenseAlphaY=on  SenseAlphaZ=on  SenseAlpha1=off  SenseAlpha2=off  SenseAlpha3=off  SenseQDDot=off  SenseRDDot=off  SenseX=on  SenseY=on  SenseZ=on  SenseRad=off  SenseAzim=off  SenseDist=off  SenseInc=off  SenseXDot=on  SenseYDot=on  SenseZDot=on  SenseRadDot=off  SenseAzimDot=off  SenseDistDot=off  SenseIncDot=off  SenseXDDot=on  SenseYDDot=on  SenseZDDot=on  SenseRadDDot=off  SenseAzimDDot=off  SenseDistDDot=off  SenseIncDDot=off
  F : PMIOPort  Port=1  Side=Right
  B : PMIOPort  Port=2  Side=Left
  Response : Outport
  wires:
  PS-Simulink Converter/1 -> Angle/1(Q)
  PS-Simulink Converter4/1 -> Mux2/4  "alphax"
  PS-Simulink Converter10/1 -> Mux1/1  "vx"
  PS-Simulink Converter12/1 -> Mux1/3  "vz"
  PS-Simulink Converter13/1 -> Mux2/1  "ax"
  PS-Simulink Converter14/1 -> Mux2/2  "ay"
  Mux/1 -> Bus Creator/1  "disp"
  Mux1/1 -> Bus Creator/2  "vel"
  Mux2/1 -> Bus Creator/3  "acc"
  Angle/1(E) -> Mux/4
  PS-Simulink Converter7/1 -> Mux/1  "x"
  PS-Simulink Converter8/1 -> Mux/2  "y"
  PS-Simulink Converter9/1 -> Mux/3  "z"
  PS-Simulink Converter5/1 -> Mux2/5  "alphay"
  PS-Simulink Converter6/1 -> Mux2/6  "alphaz"
  PS-Simulink Converter1/1 -> Mux1/4  "omegax"
  PS-Simulink Converter2/1 -> Mux1/5  "omegay"
  PS-Simulink Converter11/1 -> Mux1/2  "vy"
  PS-Simulink Converter3/1 -> Mux1/6  "omegaz"
  PS-Simulink Converter15/1 -> Mux2/3  "az"
  Bus Creator/1 -> Response/1
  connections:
  Transform Sensor/RConn1 -- F/RConn1
  B/RConn1 -- Transform Sensor/LConn1
  Transform Sensor/RConn2 -- PS-Simulink Converter/LConn1
  PS-Simulink Converter15/LConn1 -- Transform Sensor/RConn17
  PS-Simulink Converter14/LConn1 -- Transform Sensor/RConn16
  PS-Simulink Converter13/LConn1 -- Transform Sensor/RConn15
  PS-Simulink Converter12/LConn1 -- Transform Sensor/RConn14
  PS-Simulink Converter11/LConn1 -- Transform Sensor/RConn13
  PS-Simulink Converter10/LConn1 -- Transform Sensor/RConn12
  PS-Simulink Converter9/LConn1 -- Transform Sensor/RConn11
  PS-Simulink Converter8/LConn1 -- Transform Sensor/RConn10
  PS-Simulink Converter7/LConn1 -- Transform Sensor/RConn9
  PS-Simulink Converter4/LConn1 -- Transform Sensor/RConn6
  PS-Simulink Converter5/LConn1 -- Transform Sensor/RConn7
  PS-Simulink Converter6/LConn1 -- Transform Sensor/RConn8
  PS-Simulink Converter1/LConn1 -- Transform Sensor/RConn3
  PS-Simulink Converter2/LConn1 -- Transform Sensor/RConn4
  PS-Simulink Converter3/LConn1 -- Transform Sensor/RConn5

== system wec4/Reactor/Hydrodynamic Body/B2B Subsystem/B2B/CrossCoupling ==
  note: CrossCoupling block is updated by its mask initialization, which is only called on when a simulation is run. 'From' blocks are automatically created and connected based on the number of bodies in the simulation.
  Mux1 : Mux  Inputs=2
  Mux2 : Mux  Inputs=2
  vel : Outport
  acc : Outport  Port=2
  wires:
  [acc2] -> Mux2/2
  Mux2/1 -> acc/1
  [acc1] -> Mux2/1
  [vel2] -> Mux1/2
  Mux1/1 -> vel/1
  [vel1] -> Mux1/1
